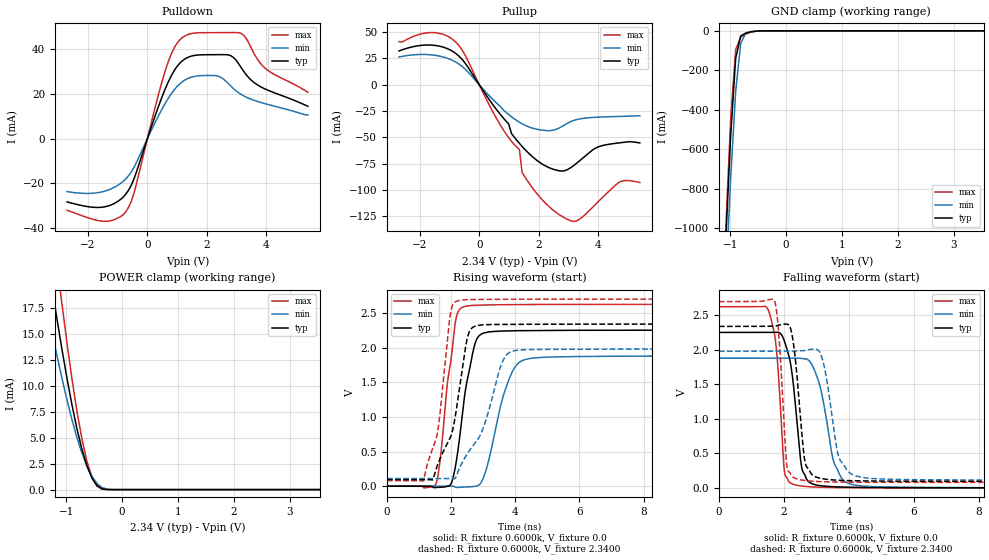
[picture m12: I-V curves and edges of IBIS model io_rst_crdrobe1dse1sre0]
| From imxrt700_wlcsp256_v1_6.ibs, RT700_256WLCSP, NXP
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[Model] io_rst_crdrobe1dse1sre0
|   Model io_rst_crdrobe1dse1sre0
| This model was characterised for following simulation conditions:
| External (pad) voltage:
|   - Typ: 2.34V,   - Min: 1.98V,   - Max: 2.7V
| Library cells for typ/min/max conditions are connected as defined below:
|  PAD_RST - External Pad
|  ipp_do - Core Input
|  ipp_obe - Output Buffer Enable
|  ASRCN3V3[3] - NC
|  ASRCN3V3[4] - NC
|  ASRCP3V3[4] - NC
|  REFAPBIAS3V3 - gnde
|  REFBAMPL3V3 - vdd1v8
|  REFCAMPH3V3 - vdd1v8
|  REFDNBIAS3V3 - vdd1v8
|  REFH3V3 - REFH3V3
|  REFL3V3 - REFL3V3
|  gnde - gnde
|  ipp_dse - vdd
|  ipp_ina235_3v - NC
|  ipp_ina40_3v - NC
|  ipp_ina_mux - NC
|  ipp_ind - NC
|  ipp_ind_1p8v - NC
|  ipp_ind_3v - NC
|  ipp_sre - gnde
|  vdd - vdd
|  vdd1v8 - vdd1v8
|  vdda - vdde3v3
|  vdde3v3 - vdde3v3
| All other pins connected to ground
Model_type I/O
Polarity   Non-Inverting
Enable   Active-High
Vinl =   0.7020V
Vinh =   1.6300V
Vmeas =  1.1700V
Cref =   15.0000pF
Rref =   0.6000k
Vref =   0.0V
C_comp   3.9956pF   3.8200pF   4.1038pF
|C_comp_pullup   0.5142pF   0.5882pF   0.4996pF
|C_comp_pulldown   2.0716pF   2.1607pF   1.8543pF
[Model Spec]
| variable   typ   min   max
Vinh   1.6300V   NA   NA
Vinl   0.7020V   NA   NA
Vref   0.0V   0.0V   0.0V
Cref   15.0000pF   15.0000pF   15.0000pF
Rref   0.6000k   0.6000k   0.6000k
[Receiver Thresholds]
Vcross_high  =   0.0V
Vcross_low  =   0.0V
Vdiff_ac  =   0.0V
Vdiff_dc  =   0.0V
Tdiffslew_ac  =   0.0S
[Temperature Range]   25.0000   0.1250k   -40.0000
[Voltage Range]   2.3400V   1.9800V   2.7000V
[Pullup Reference]   2.3400V   1.9800V   2.7000V
[Pulldown Reference]   0.0V   0.0V   0.0V
[POWER Clamp Reference]   2.3400V   1.9800V   2.7000V
[GND Clamp Reference]   0.0V   0.0V   0.0V
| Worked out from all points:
|   slope of the pulldown table from 0 to 0.351 V, typ, clamps not added: 25.9 ohm
|   slope of the pullup table from 0 to 0.351 V, typ, clamps not added: 23.9 ohm
|   GND clamp passes 1 mA (typ) near -0.49 V on its own axis
|   POWER clamp passes 1 mA (typ) near -0.53 V on its own axis
|   rising waveform, R_fixture 0.6000k, V_fixture 0.0: 20-80 % time 429ps typ, 602ps min, 368ps max; typ from 0 V to 2.25 V
|   rising waveform, R_fixture 0.6000k, V_fixture 2.3400: 20-80 % time 607ps typ, 936ps min, 427ps max; typ from 0.094 V to 2.34 V
|   falling waveform, R_fixture 0.6000k, V_fixture 0.0: 20-80 % time 299ps typ, 443ps min, 222ps max; typ from 2.25 V to 0 V
|   falling waveform, R_fixture 0.6000k, V_fixture 2.3400: 20-80 % time 254ps typ, 362ps min, 194ps max; typ from 2.34 V to 0.094 V
[Pulldown]
|Voltage   I(typ)   I(min)   I(max)
-2.7V     -28.24mA   -23.64mA   -31.98mA
-1.44V    -30.44mA   -23.46mA   -36.9mA
-720mV    -24.64mA   -17.86mA   -32.55mA
-450mV    -17.94mA   -12.78mA   -24.31mA
630mV     23.17mA    16.47mA    31.53mA
900mV     30.36mA    21.79mA    40.52mA
1.26V     35.6mA     26.18mA    45.89mA
2.34V     37.55mA    28.09mA    47.4mA
2.79V     37.18mA    23.72mA    47.41mA
3.15V     31.9mA     19.83mA    47.08mA
3.96V     22.22mA    15.65mA    31.51mA
5.4V      14.48mA    10.63mA    20.78mA
[Pullup]
|Voltage   I(typ)   I(min)   I(max)
-2.7V     32.17mA    26.42mA    41.08mA
-1.53V    37.55mA    28.2mA     49.59mA
-720mV    28.16mA    20.36mA    38.44mA
630mV     -25.37mA   -18.65mA   -34.47mA
1.35V     -55.63mA   -35.58mA   -61.51mA
1.44V     -58.52mA   -37.05mA   -83.28mA
2.16V     -76.03mA   -43.22mA   -110.5mA
2.88V     -81.56mA   -38mA      -126.6mA
3.33V     -73.2mA    -32.68mA   -128.5mA
4.05V     -58.5mA    -30.69mA   -109.7mA
4.77V     -54.97mA   -30mA      -91.76mA
5.4V      -55.22mA   -29.39mA   -92.85mA
[GND_clamp]
|Voltage   I(typ)   I(min)   I(max)
-2.7V     -12.91A    -12.88A    -13.56A
-1.08V    -1.077A    -1.286A    -1.025A
-990mV    -533.6mA   -749.4mA   -449.1mA
-900mV    -139.2mA   -307mA     -94.25mA
-810mV    -25.49mA   -63.91mA   -32.87mA
-720mV    -11.78mA   -11.41mA   -16.65mA
-540mV    -1.684mA   -1.901mA   -2.149mA
-360mV    -36.04uA   -133.3uA   -15.05uA
5.4V      0A         0A         0A
[POWER_clamp]
|Voltage   I(typ)   I(min)   I(max)
-2.7V     73.96mA    57.58mA    95.4mA
-1.44V    26.15mA    20.18mA    34.67mA
-1.35V    22.86mA    17.7mA     30.34mA
-1.26V    19.66mA    15.3mA     26.09mA
-1.17V    16.56mA    12.98mA    21.97mA
-1.08V    13.59mA    10.78mA    17.99mA
-900mV    8.212mA    6.776mA    10.73mA
-720mV    3.9mA      3.518mA    4.888mA
-630mV    2.284mA    2.252mA    2.724mA
-540mV    1.103mA    1.268mA    1.195mA
-360mV    77.93uA    204.3uA    41.52uA
5.4V      0A         0A         0A
[Ramp]
| variable   typ   min   max
dV/dt_r  1.3518/0.4294n   1.1288/0.6015n   1.5754/0.3683n
dV/dt_f  1.3475/0.2544n   1.1218/0.3624n   1.5719/0.1937n
R_load = 0.6000k
[Rising Waveform]
R_fixture= 0.6000k
V_fixture= 0.0
V_fixture_min= 0.0
V_fixture_max= 0.0
|time   V(typ)   V(min)   V(max)
0s        54.47nV    1.425uV    18.12nV
1.523ns   -19.62mV   -588.5uV   28.19mV
1.661ns   -16.4mV    -639.9uV   392.8mV
1.976ns   19.12mV    -209.9uV   1.767V
2.147ns   320.5mV    -18.67mV   2.407V
2.623ns   1.808V     -9.312mV   2.608V
3.029ns   2.212V     150.7mV    2.615V
3.906ns   2.243V     1.652V     2.621V
4.684ns   2.247V     1.854V     2.623V
60ns      2.253V     1.881V     2.626V
[Rising Waveform]
R_fixture= 0.6000k
V_fixture= 2.3400
V_fixture_min= 1.9800
V_fixture_max= 2.7000
|time   V(typ)   V(min)   V(max)
0s        94.13mV    110.3mV    80.1mV
1.137ns   93.59mV    110.2mV    81.94mV
1.587ns   320.7mV    109.7mV    811.5mV
1.993ns   726.1mV    110.4mV    2.532V
2.362ns   1.742V     356.6mV    2.688V
2.673ns   2.292V     579.2mV    2.694V
3.028ns   2.33V      876.7mV    2.696V
3.651ns   2.335V     1.845V     2.698V
4.211ns   2.337V     1.968V     2.699V
60ns      2.34V      1.98V      2.7V
[Falling Waveform]
R_fixture= 0.6000k
V_fixture= 0.0
V_fixture_min= 0.0
V_fixture_max= 0.0
|time   V(typ)   V(min)   V(max)
0s        2.253V     1.881V     2.626V
1.515ns   2.254V     1.881V     2.582V
1.758ns   2.253V     1.881V     2.061V
1.936ns   2.212V     1.881V     815.7mV
2.042ns   2.089V     1.882V     179.6mV
2.666ns   160mV      1.87V      20.27mV
3.088ns   33.93mV    1.512V     9.299mV
3.556ns   15.54mV    346.6mV    4.543mV
4.514ns   5.702mV    23.66mV    1.342mV
60ns      1.229uV    6.675uV    688.5nV
[Falling Waveform]
R_fixture= 0.6000k
V_fixture= 2.3400
V_fixture_min= 1.9800
V_fixture_max= 2.7000
|time   V(typ)   V(min)   V(max)
0s        2.34V      1.98V      2.7V
1.71ns    2.344V     1.98V      2.712V
1.853ns   2.361V     1.979V     2.162V
2.079ns   2.374V     1.981V     375mV
2.174ns   2.348V     1.982V     226.6mV
2.767ns   267.9mV    2.004V     100.2mV
3.187ns   132mV      1.862V     89.2mV
3.738ns   109mV      393.9mV    83.92mV
4.771ns   99.13mV    134.2mV    81.13mV
60ns      94.14mV    110.3mV    80.1mV
